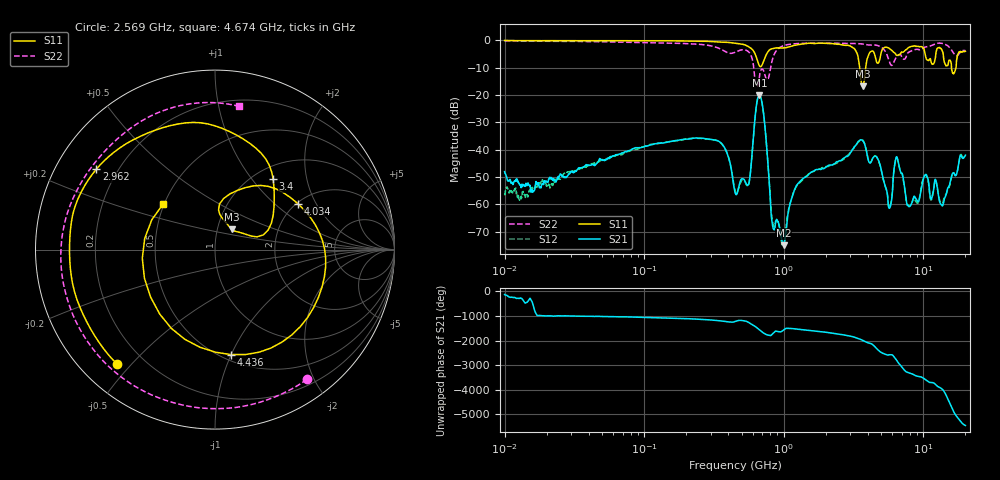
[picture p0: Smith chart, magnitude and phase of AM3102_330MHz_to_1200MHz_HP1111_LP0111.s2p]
! Date/Time: Tue, Sep 11, 2018 5:24 PM
! Network Analyzer: Agilent Technologies E8362B Rev: A.07.50.63
! Sweep from 0.010 to 20.000 GHz, 1601 Points, Sweep Type: LOG
! Power Supply: 4.949 V, 0.001 A
# Hz S DB R 50
!freq MagS11 AngS11 MagS21 AngS21 MagS12 AngS12 MagS22 AngS22
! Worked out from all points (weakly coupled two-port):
!   1601 points, 10 MHz to 20 GHz, reference 50 ohm
!   highest |S21| = -20.00 dB at 669.7 MHz (marker M1); lowest = -75.0 dB at 998.1 MHz (marker M2)
!   lowest |S11| = -16.7 dB at 3.668 GHz (marker M3), VSWR 1.34, Z = 58.5 + j13.5 ohm
!   |S11| at or under -10 dB: 3.498 GHz to 3.863 GHz (364.6 MHz wide, 9.91 % of centre); 15.91 GHz to 17.11 GHz (1.204 GHz wide, 7.29 % of centre)
!   |S22| runs from -16.9 to -0.2 dB; largest |S21 - S12| = 0.0049
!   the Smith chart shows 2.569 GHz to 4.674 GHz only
!   S11 on the Smith chart (normalised r, x): 2.569 GHz: 0.11, -0.45; 2.962 GHz: 0.12, +0.30; 3.4 GHz: 1.21, +1.28; 4.034 GHz: 2.03, +1.44; 4.436 GHz: 0.55, -1.00; 4.674 GHz: 0.49, +0.30
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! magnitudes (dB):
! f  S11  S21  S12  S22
! 10 MHz  0.0  -48.0  -56.1  -0.2
! 35.55 MHz  -0.1  -46.6  -46.8  -0.4
! 126.4 MHz  -0.2  -37.6  -37.7  -0.9
! 342.8 MHz  -0.6  -36.9  -37.0  -2.9
! 447.2 MHz  -1.0  -55.6  -55.0  -4.3
! 559.1 MHz  -2.3  -52.6  -52.9  -4.2
! 669.7 MHz  -9.3  -20.0  -20.0  -13.1
! 833.3 MHz  -3.0  -68.1  -66.6  -6.6
! 998.1 MHz  -2.7  -75.0  -74.7  -1.9
! 1.59 GHz  -1.1  -48.1  -48.1  -1.0
! 2.569 GHz  -1.5  -44.0  -44.0  -1.0
! 2.962 GHz  -2.0  -41.7  -41.4  -1.1
! 3.4 GHz  -5.9  -37.1  -37.3  -1.2
! 3.668 GHz  -16.7  -36.7  -36.4  -1.3
! 4.034 GHz  -5.6  -43.9  -43.7  -1.7
! 4.436 GHz  -4.6  -42.5  -42.4  -1.7
! 4.674 GHz  -8.3  -43.0  -43.1  -1.8
! 5.652 GHz  -2.8  -61.2  -60.8  -7.1
! 6.426 GHz  -5.4  -42.6  -42.9  -6.0
! 7.845 GHz  -2.7  -60.7  -60.4  -4.3
! 13.55 GHz  -3.3  -60.3  -59.5  -1.1
! 20 GHz  -4.0  -42.0  -42.4  -3.7
